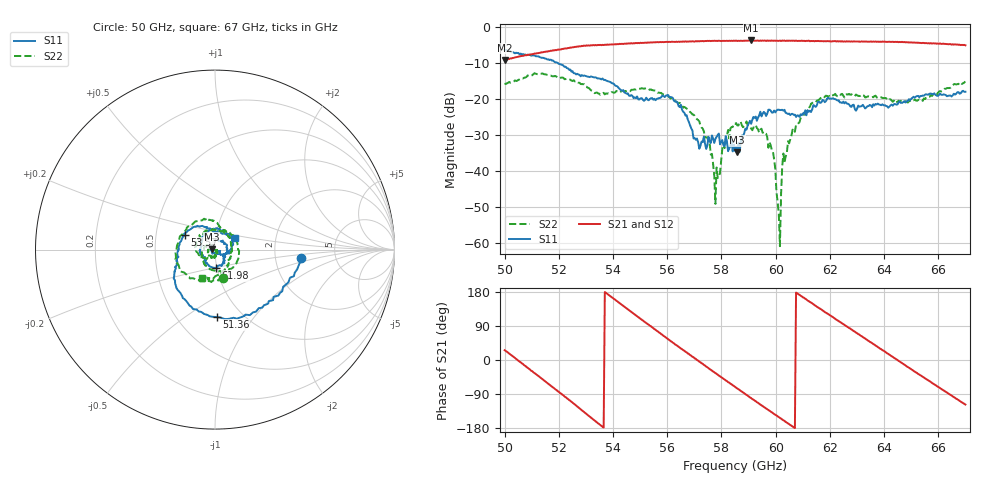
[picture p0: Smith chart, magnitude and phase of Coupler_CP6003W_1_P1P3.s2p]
!Agilent Technologies,E8361A,US42410132,A.06.03.05
!Agilent E8361A: A.06.03.05
!Date: Friday, July 11, 2008 16:42:56
!Correction: S11(Full 2 Port(1,2)) S21(Full 2 Port(1,2)) S12(Full 2 Port(1,2)) S22(Full 2 Port(1,2))
!S2P File: Measurements: S11, S21, S12, S22:
# Hz S  MA  R 50
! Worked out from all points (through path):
!   401 points, 50 GHz to 67 GHz, reference 50 ohm
!   highest |S21| = -3.71 dB at 59.09 GHz (marker M1); lowest = -9.1 dB at 50 GHz (marker M2)
!   group delay of S21, straight-line fit = 141 ps
!   lowest |S11| = -34.8 dB at 58.59 GHz (marker M3), VSWR 1.04, Z = 48.2 + j0.0602 ohm
!   |S11| at or under -10 dB: 51.97 GHz to end of sweep
!   |S22| runs from -60.9 to -12.8 dB; largest |S21 - S12| = 0.011
!   S11 on the Smith chart (normalised r, x): 50 GHz: 2.81, -0.35; 51.36 GHz: 0.77, -0.67; 53.57 GHz: 0.70, +0.12; 61.98 GHz: 0.99, -0.20; 67 GHz: 1.24, +0.16
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5e10  0.4818 -5.8  0.3497 25.8  0.3535 26.1  0.1661 -74.0
5.136e10  0.3757 -88.5  0.4463 -48.5  0.447 -49.0  0.2254 -164.3
5.28475e10  0.2155 -169.4  0.549 -132.4  0.5477 -132.4  0.1616 95.0
5.357e10  0.1878 154.4  0.5613 -173.6  0.5707 -173.9  0.1194 64.3
5.476e10  0.1029 96.7  0.5979 122.5  0.5994 122.4  0.1352 -9.2
5.5695e10  0.1032 58.9  0.6162 72.6  0.6194 73.0  0.1233 -79.9
5.64175e10  0.08016 -3.3  0.6292 35.1  0.6236 34.8  0.08816 -144.3
5.70975e10  0.0283 -49.5  0.6346 0.1  0.6335 0.7  0.05257 156.0
5.782e10  0.02996 -51.4  0.6451 -36.7  0.6435 -36.4  0.01121 -11.1
5.85e10  0.01908 -173.5  0.6432 -70.7  0.6484 -70.4  0.04521 -92.5
5.8585e10  0.01819 178.0  0.6413 -75.2  0.6514 -74.8  0.04309 -99.9
5.9095e10  0.04533 93.7  0.6523 -100.4  0.6546 -100.7  0.03912 -145.4
5.986e10  0.06493 13.3  0.6517 -138.4  0.6456 -138.4  0.0194 144.0
6.0115e10  0.07121 -9.7  0.6437 -150.8  0.6467 -150.7  0.002561 -15.8
6.03275e10  0.07102 -18.6  0.6495 -160.8  0.6509 -160.9  0.01332 -57.2
6.054e10  0.05983 -30.5  0.6441 -171.6  0.6437 -171.7  0.02776 -76.4
6.13475e10  0.07163 -48.6  0.6393 149.4  0.6435 149.3  0.08826 -149.3
6.1985e10  0.1014 -86.4  0.6359 118.8  0.6411 118.7  0.111 166.8
6.3005e10  0.07376 -142.5  0.6312 70.8  0.6318 70.9  0.1128 96.5
6.4195e10  0.07859 164.7  0.6252 14.0  0.6274 14.1  0.09953 21.4
6.5725e10  0.1192 84.2  0.5985 -58.0  0.6012 -58.2  0.1141 -48.8
6.7e10  0.1265 29.9  0.5584 -117.6  0.5535 -117.9  0.1755 -113.7
